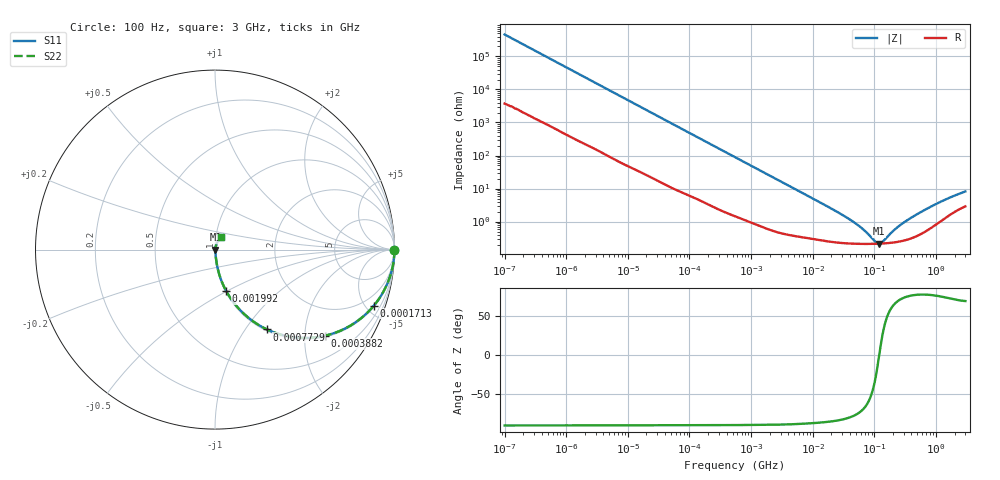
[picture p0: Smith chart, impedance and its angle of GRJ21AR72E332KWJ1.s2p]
!Murata Part Number: GRJ21AR72E332KWJ1
!These Parameters are Measured in Series Mode Connection
!Data Generated on Jun 19, 2026
!  o--ll--o
!Port1  Port2
!  o------o
!Operation Temp=25[degC], DC Bias Voltage=0[V]
!Freq. Start=100[Hz] Stop=3[GHz] 401[Steps]
# Hz S RI R 50
!Freq.(Hz) S11(Real) S11(Imag) S21(Real) S21(Imag) S12(Real) S12(Imag) S22(Real) S22(Imag)
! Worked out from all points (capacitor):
!   401 points, 100 Hz to 3 GHz, reference 50 ohm
!   read as one part in series: C = 3.44 nF near 109 Hz
!   lowest |Z| = 215 mohm at 118.9 MHz (marker M1)
!   series resonance near 119.7 MHz, so ESL is about 510 pH
!   S11 on the Smith chart (normalised r, x): 100 Hz: open; 171.3 kHz: 1.08, -5.65; 388.2 kHz: 1.04, -2.51; 772.9 kHz: 1.02, -1.27; 1.992 MHz: 1.01, -0.50; 3 GHz: 1.06, +0.15
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100  1 -0.000217  1.8e-06 0.000217  1.8e-06 0.000217  1 -0.000217
1788  0.9999 -0.00381  5.02e-05 0.00381  5.02e-05 0.00381  0.9999 -0.00381
31977  0.9948 -0.0664  0.00516 0.0664  0.00516 0.0664  0.9948 -0.0664
75630  0.9741 -0.1528  0.0259 0.1528  0.0259 0.1528  0.9741 -0.1528
171338  0.8855 -0.3117  0.1145 0.3117  0.1145 0.3117  0.8855 -0.3117
388167  0.6104 -0.4803  0.3896 0.4803  0.3896 0.4803  0.6104 -0.4803
547723  0.4443 -0.4888  0.5557 0.4888  0.5557 0.4888  0.4443 -0.4888
772864  0.2905 -0.4451  0.7095 0.4451  0.7095 0.4451  0.2905 -0.4451
1188587  0.1516 -0.3488  0.8484 0.3488  0.8484 0.3488  0.1516 -0.3488
1992254  0.0628 -0.2315  0.9372 0.2315  0.9372 0.2315  0.0628 -0.2315
4141163  0.018 -0.1175  0.982 0.1175  0.982 0.1175  0.018 -0.1175
9794414  0.00557 -0.0506  0.9944 0.0506  0.9944 0.0506  0.00557 -0.0506
4.418008e7  0.00224 -0.00997  0.9978 0.00997  0.9978 0.00997  0.00224 -0.00997
6.794454e7  0.00213 -0.00509  0.9979 0.00509  0.9979 0.00509  0.00213 -0.00509
1.044919e8  0.00212 -0.00116  0.9979 0.00116  0.9979 0.00116  0.00212 -0.00116
1.188943e8  0.00214 -5.76e-05  0.9979 5.76e-05  0.9979 5.76e-05  0.00214 -5.76e-05
1.352818e8  0.00217 0.00105  0.9978 -0.00105  0.9978 -0.00105  0.00217 0.00105
1.751444e8  0.00226 0.00332  0.9977 -0.00332  0.9977 -0.00332  0.00226 0.00332
2.812011e8  0.00264 0.00816  0.9974 -0.00816  0.9974 -0.00816  0.00264 0.00816
5.59889e8  0.00445 0.0186  0.9955 -0.0186  0.9955 -0.0186  0.00445 0.0186
1.382454e9  0.0141 0.0426  0.9859 -0.0426  0.9859 -0.0426  0.0141 0.0426
3e9  0.0334 0.0718  0.9666 -0.0718  0.9666 -0.0718  0.0334 0.0718
